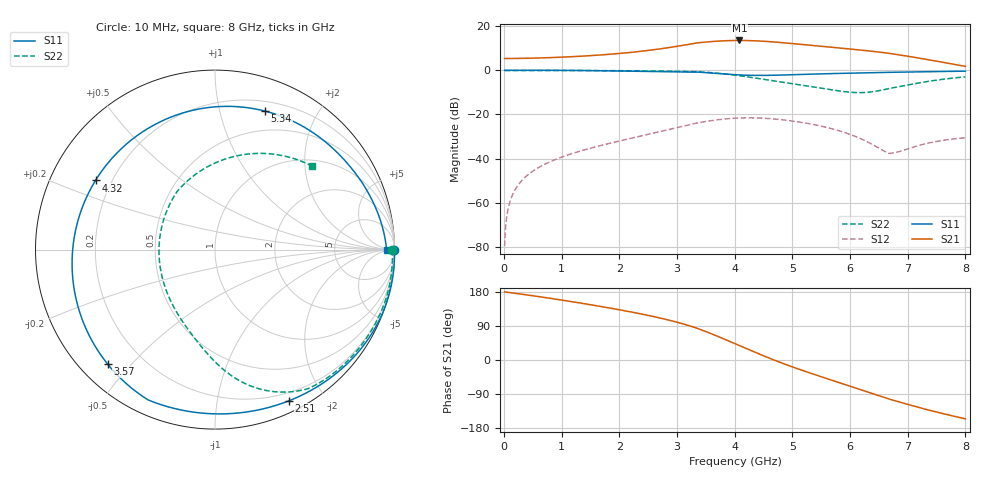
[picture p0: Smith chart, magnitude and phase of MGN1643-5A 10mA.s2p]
! Port[1] = GATE
! Port[2] = DRAIN
! [Type]  S-parameter s2p file touchstone ver. 1.0
! [Object]  MGN1643-5A
! [Bias]  10 mA
! [Version]  1.0
! [Date]  Thu May 19 11:03:42 2026
! [Source]  This file was created in JSC "ICC Milandr".
! [Disclaimer] Property of JSC "ICC Milandr". Unauthorized reproduction and/or distribution is strictly prohibited.
!  The file and the data are provided "AS IS" and with all faults and disclaim all warranties, express and implied, including
!  without limitation any implied warranties of merchantability, fitness for a particular purpose.
!  JSC "ICC Milandr" assumes no liability for:
!  1) the accuracy of the data provided;
!  2) the proper functioning of this data;
!  3) infringement of patents, copyrights or intellectual property rights resulting from the use of this data.
!  JSC "ICC Milandr" reserves the right to make changes to the products and the data without prior notice.
!  Please, be aware that your receipt and use of the file provided shall serve as acceptance of these terms and conditions.
!  If you do not accept these terms, you should return or destroy this file and any other accompanying information immediately.
# Hz S MA R 12.5
! freq  S11mag  S11ang  S21mag  S21ang  S12mag  S12ang  S22mag  S22ang
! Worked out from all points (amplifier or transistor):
!   800 points, 10 MHz to 8 GHz, reference 12.5 ohm
!   highest |S21| = 13.5 dB at 4.08 GHz (marker M1)
!   |S21| within 3 dB of that: 2.919 GHz to 5.648 GHz (2.729 GHz wide, 63.7 % of centre)
!   unconditionally stable (mu >= 1): 6.026 GHz to 7.457 GHz
!   at 1.34 GHz: K = 0.17, MSG = 21.4 dB, |S12| = -36.5 dB
!   at 4.01 GHz: K = 0.43, MSG = 17.6 dB, |S12| = -21.7 dB
!   at 8 GHz: K = 0.64, MSG = 16.2 dB, |S12| = -30.6 dB
!   S11 on the Smith chart (normalised r, x): 10 MHz: open; 2.51 GHz: 0.11, -1.59; 3.57 GHz: 0.08, -0.43; 4.32 GHz: 0.14, +0.26; 5.34 GHz: 0.29, +1.38; 8 GHz: 45, -2
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1e7  1 -0.2  1.853 179.8  0.0001032 86.9  0.9884 -0.1
1.1e8  1.001 -2.2  1.856 177.8  0.001127 87.8  0.9893 -1.4
3.1e8  1.002 -6.1  1.869 173.6  0.003191 84.7  0.9907 -4.0
1.35e9  0.9908 -28.4  2.095 149.7  0.01516 65.3  0.9897 -17.9
2.51e9  0.9376 -64.0  2.837 117.3  0.03557 37.6  0.9692 -36.6
2.68e9  0.9286 -71.6  3.031 111.7  0.04 32.5  0.9645 -39.9
3.16e9  0.9133 -99.7  3.796 92.8  0.05615 15.0  0.9445 -51.2
3.36e9  0.9133 -115.5  4.208 83.0  0.0646 5.6  0.9282 -57.0
3.57e9  0.8743 -133.2  4.459 70.8  0.07169 -5.5  0.8897 -63.1
3.79e9  0.8324 -154.2  4.656 57.1  0.07799 -17.9  0.8376 -69.7
4.01e9  0.7966 -177.1  4.75 42.7  0.08224 -30.6  0.7755 -76.3
4.08e9  0.7877 175.4  4.756 38.1  0.08306 -34.7  0.7543 -78.3
4.32e9  0.7691 149.9  4.687 22.5  0.08369 -48.2  0.6803 -85.1
4.52e9  0.7676 129.9  4.545 9.8  0.08182 -58.8  0.6208 -90.4
4.74e9  0.7766 110.3  4.331 -3.4  0.07771 -69.4  0.5608 -96.3
5.04e9  0.7978 87.9  4.001 -20.3  0.0697 -82.2  0.4887 -105.5
5.34e9  0.8205 70.1  3.675 -36.1  0.05993 -93.0  0.4249 -117.5
5.65e9  0.8415 55.6  3.365 -51.7  0.04873 -102.2  0.3663 -135.0
5.98e9  0.861 43.4  3.061 -68.0  0.03609 -109.2  0.3208 -162.1
6.67e9  0.9009 24.4  2.437 -102.7  0.0131 -89.5  0.3868 123.0
7.26e9  0.9289 13.0  1.831 -127.9  0.02088 -61.0  0.536 77.0
8e9  0.9563 -0.1  1.228 -155.2  0.02956 -70.7  0.7127 40.8
